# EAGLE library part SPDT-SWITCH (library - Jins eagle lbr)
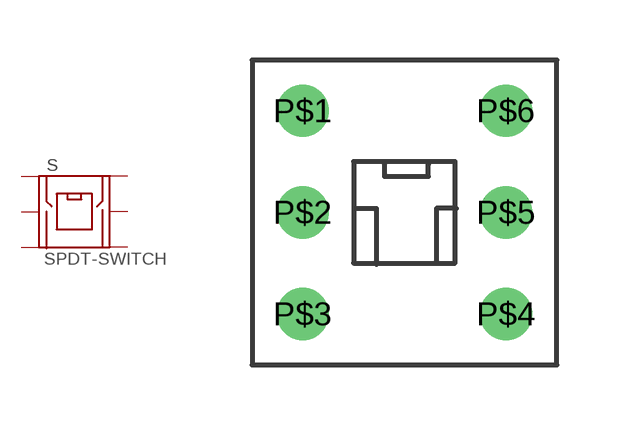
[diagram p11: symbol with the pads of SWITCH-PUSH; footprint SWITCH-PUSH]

Designator prefix S

## SPDT-SWITCH-8.5MM  [SWITCH-PUSH]
P$1  1
P$2  2
P$3  3
P$4  4
P$5  5
P$6  6

## Footprint SWITCH-PUSH (pad centres in mm)
drill 0.8: P$1 -2.54,2.54; P$2 -2.54,0; P$3 -2.54,-2.54; P$4 2.54,-2.54; P$5 2.54,0; P$6 2.54,2.54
